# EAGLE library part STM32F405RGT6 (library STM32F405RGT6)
MCU 32-Bit, ARM Cortex M4, 1MB Flash STMicroelectronics STM32F405RGT6, 32bit ARM Cortex M4F Microcontroller, 168MHz, 1024 kB Flash, 64-Pin LQFP Source: Datasheet
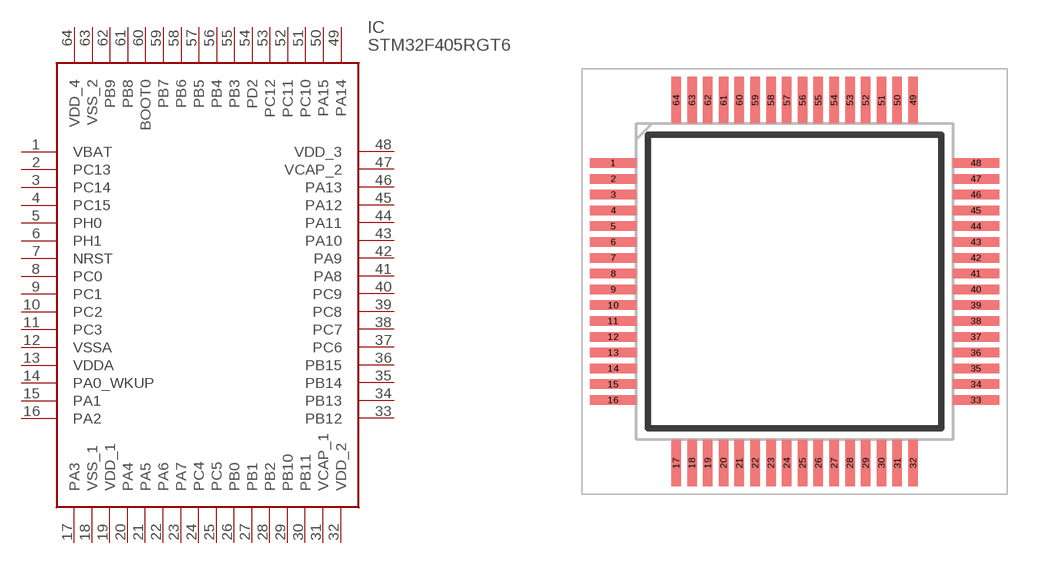
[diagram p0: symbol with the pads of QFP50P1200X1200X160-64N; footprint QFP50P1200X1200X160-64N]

Designator prefix IC

## STM32F405RGT6 (Arrow_Part_Number: STM32F405RGT6; Arrow_Price-Stock: https://www.arrow.com/en/products/stm32f405rgt6/stmicroelectronics; Description: MCU 32-Bit, ARM Cortex M4, 1MB Flash STMicroelectronics STM32F405RGT6, 32bit ARM Cortex M4F Microcontroller, 168MHz, 1024 kB Flash, 64-Pin LQFP; Height: 1.6mm; Manufacturer_Name: STMicroelectronics; Manufacturer_Part_Number: STM32F405RGT6; Mouser_Part_Number: 511-STM32F405RGT6; Mouser_Price-Stock: https://www.mouser.co.uk/ProductDetail/STMicroelectronics/STM32F405RGT6?qs=Z8%252BeY1k3TIKgj7QWsYGpQw%3D%3D)  [QFP50P1200X1200X160-64N]
1  VBAT
2  PC13
3  PC14
4  PC15
5  PH0
6  PH1
7  NRST
8  PC0
9  PC1
10  PC2
11  PC3
12  VSSA
13  VDDA
14  PA0_WKUP
15  PA1
16  PA2
17  PA3
18  VSS_1
19  VDD_1
20  PA4
21  PA5
22  PA6
23  PA7
24  PC4
25  PC5
26  PB0
27  PB1
28  PB2
29  PB10
30  PB11
31  VCAP_1
32  VDD_2
33  PB12
34  PB13
35  PB14
36  PB15
37  PC6
38  PC7
39  PC8
40  PC9
41  PA8
42  PA9
43  PA10
44  PA11
45  PA12
46  PA13
47  VCAP_2
48  VDD_3
49  PA14
50  PA15
51  PC10
52  PC11
53  PC12
54  PD2
55  PB3
56  PB4
57  PB5
58  PB6
59  PB7
60  BOOT0
61  PB8
62  PB9
63  VSS_2
64  VDD_4

## Footprint QFP50P1200X1200X160-64N (pad centres in mm)
LQFP - 64 pin, 10 x 10 mm
smd 1.475 x 0.3: 1 -5.738,3.75; 2 -5.738,3.25; 3 -5.738,2.75; 4 -5.738,2.25; 5 -5.738,1.75; 6 -5.738,1.25; 7 -5.738,0.75; 8 -5.738,0.25; 9 -5.738,-0.25; 10 -5.738,-0.75; 11 -5.738,-1.25; 12 -5.738,-1.75; 13 -5.738,-2.25; 14 -5.738,-2.75; 15 -5.738,-3.25; 16 -5.738,-3.75; 33 5.738,-3.75; 34 5.738,-3.25; 35 5.738,-2.75; 36 5.738,-2.25; 37 5.738,-1.75; 38 5.738,-1.25; 39 5.738,-0.75; 40 5.738,-0.25; 41 5.738,0.25; 42 5.738,0.75; 43 5.738,1.25; 44 5.738,1.75; 45 5.738,2.25; 46 5.738,2.75; 47 5.738,3.25; 48 5.738,3.75
smd 0.3 x 1.475: 17 -3.75,-5.738; 18 -3.25,-5.738; 19 -2.75,-5.738; 20 -2.25,-5.738; 21 -1.75,-5.738; 22 -1.25,-5.738; 23 -0.75,-5.738; 24 -0.25,-5.738; 25 0.25,-5.738; 26 0.75,-5.738; 27 1.25,-5.738; 28 1.75,-5.738; 29 2.25,-5.738; 30 2.75,-5.738; 31 3.25,-5.738; 32 3.75,-5.738; 49 3.75,5.738; 50 3.25,5.738; 51 2.75,5.738; 52 2.25,5.738; 53 1.75,5.738; 54 1.25,5.738; 55 0.75,5.738; 56 0.25,5.738; 57 -0.25,5.738; 58 -0.75,5.738; 59 -1.25,5.738; 60 -1.75,5.738; 61 -2.25,5.738; 62 -2.75,5.738; 63 -3.25,5.738; 64 -3.75,5.738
